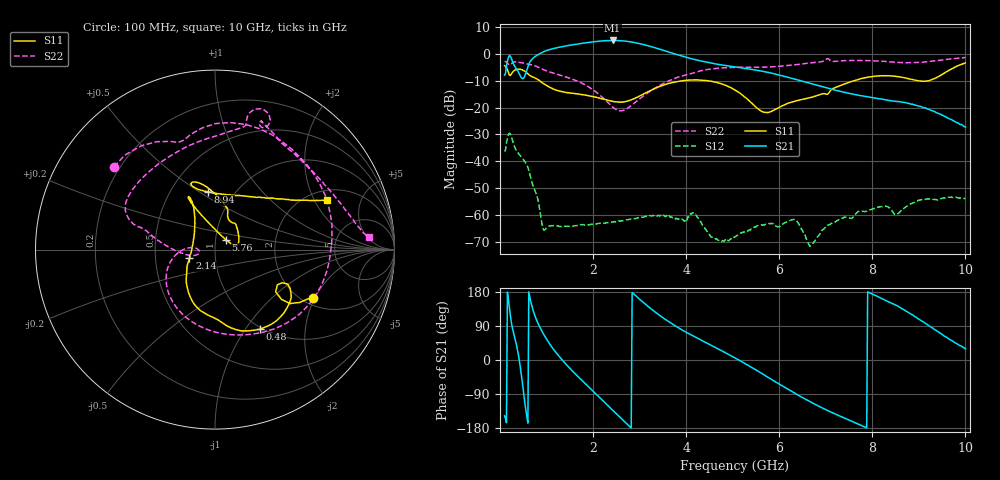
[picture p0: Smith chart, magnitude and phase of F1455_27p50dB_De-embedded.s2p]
! Integrated Device Technology
! Corporate Headquarters
! 6024 Silver Creek Valley Road
! San Jose, CA 95138  USA
! Phone:  1-408-284-8200
! Toll Free:  1-800-223-1366
! Webpage:  http://www.idt.com/
! Timing and RF Division
! 515 Groton Road, Suite 102
! Westford, MA 01886-6024
! Device:  F1455
! Description: 6-bit 0.5 dB Transmit Variable Gain Amplifier
! Frequency:  1400.0 -  2300.00 MHz
! Package:  6x6 mm Thin QFN Plastic Package: 28 pin
! State:  55
! Atten State:  27.5 dB
! Voltage:  +5.00 Volts
! Current:  217.607 mA
! Data:  The device was measured on a the F1455 evaluation board which has
!  individual transmission lines to the RF pins.  Data was collected
!  using a calibrated network analyzer.  The evaluation board was
!  de-embedded using a TRL calibration technique.
!  The reference plane is the edge of the package pin.
!  Pin  1 = CSb
!  Pin  2 = DATA
!  Pin  3 = CLK
!  Pin  4 = RSET
!  Pin  5 = GND
!  Pin  6 = RFIN  = Port 1
!  Pin  7 = GND
!  Pin  8 = NC
!  Pin  9 = NC
!  Pin 10 = NC
!  Pin 11 = NC
!  Pin 12 = NC
!  Pin 13 = NC
!  Pin 14 = /STBY
!  Pin 15 = GND
!  Pin 16 = RFOUT  = Port 2
!  Pin 17 = GND
!  Pin 18 = NC
!  Pin 19 = NC
!  Pin 20 = NC
!  Pin 21 = GND
!  Pin 22 = NC
!  Pin 23 = GND
!  Pin 24 = NC
!  Pin 25 = NC
!  Pin 26 = NC
!  Pin 27 = GND
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# GHz S dB R 50
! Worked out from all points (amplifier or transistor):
!   496 points, 100 MHz to 10 GHz, reference 50 ohm
!   highest |S21| = 5.1 dB at 2.42 GHz (marker M1)
!   |S21| within 3 dB of that: 1.155 GHz to 3.385 GHz (2.23 GHz wide, 98.3 % of centre)
!   unconditionally stable (mu >= 1): start of sweep to end of sweep
!   at 1.74 GHz: K = 422.67, MAG = 4.5 dB, |S12| = -63.6 dB
!   at 5.06 GHz: K = 1443.57, MAG = -2.9 dB, |S12| = -68.2 dB
!   at 10 GHz: K = 774.81, MAG = -18.5 dB, |S12| = -53.9 dB
!   S11 on the Smith chart (normalised r, x): 100 MHz: 2.27, -1.94; 480 MHz: 0.97, -1.17; 2.14 GHz: 0.75, -0.07; 5.76 GHz: 1.12, +0.12; 8.94 GHz: 0.75, +0.54; 10 GHz: 2.43, +2.56
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0.1  -4.30 -26.1  -7.85 -147.1  -36.38 47.5  -2.75 140.7
0.18  -6.70 -36.8  -1.31 161.2  -30.15 -6.4  -3.71 112.5
0.26  -6.98 -25.3  -2.28 89.1  -31.64 -77.2  -3.33 96.0
0.38  -5.65 -42.7  -6.18 24.7  -36.65 -118.5  -3.00 58.2
0.48  -5.87 -60.7  -9.15 -58.5  -38.84 -150.4  -3.25 31.7
0.66  -8.17 -88.0  -2.50 155.5  -46.06 139.9  -3.94 -10.3
0.78  -9.11 -103.1  -0.61 107.5  -52.15 115.7  -4.54 -37.1
0.94  -11.05 -121.9  0.90 67.7  -65.67 119.3  -5.83 -67.5
1.32  -13.98 -141.8  2.75 2.6  -64.38 118.3  -8.01 -119.0
1.76  -15.07 -151.2  4.02 -53.8  -63.74 86.4  -10.83 -157.6
2.14  -16.43 -161.2  4.85 -98.7  -63.21 71.3  -15.19 179.6
2.42  -17.60 -177.1  5.11 -132.1  -62.65 64.5  -19.73 176.4
2.82  -17.08 146.4  4.55 -179.5  -61.58 53.6  -19.22 -164.1
3.4  -12.29 118.6  2.02 120.6  -60.11 31.8  -12.03 177.7
4.08  -9.67 116.1  -1.57 68.1  -59.85 19.0  -7.37 163.4
5.06  -13.48 111.9  -4.80 4.9  -68.17 39.4  -4.94 148.4
5.76  -21.80 41.8  -6.81 -45.7  -63.34 30.7  -4.81 119.1
6.34  -17.55 14.3  -9.36 -88.1  -61.73 -13.6  -3.97 89.6
6.7  -16.10 34.4  -11.10 -112.4  -71.23 -167.9  -3.23 78.6
8.36  -8.08 109.5  -17.30 152.8  -57.35 66.7  -2.84 62.6
8.94  -9.77 97.1  -19.13 113.1  -54.91 78.7  -3.16 39.1
10  -3.29 24.0  -27.20 29.3  -53.95 12.7  -1.28 4.7
